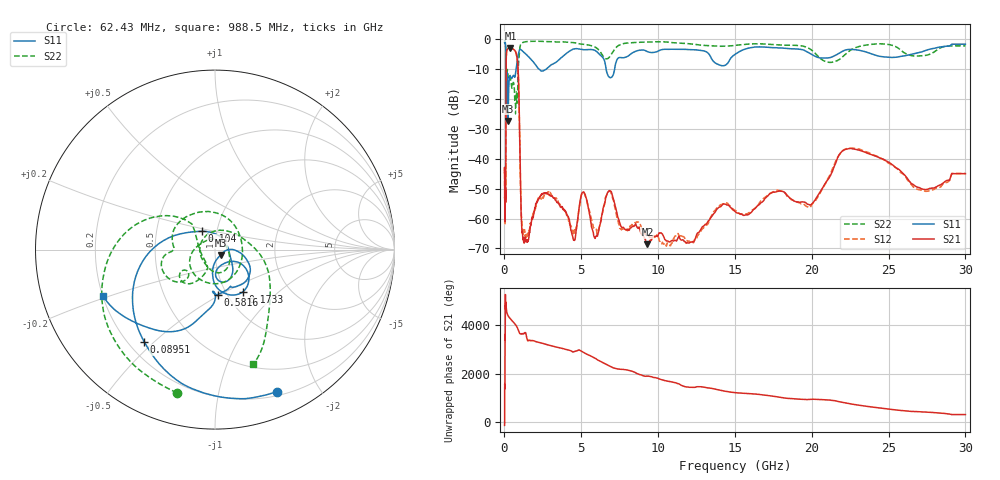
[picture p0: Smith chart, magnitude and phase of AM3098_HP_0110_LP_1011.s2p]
! Date/Time: Thu, Feb 28, 2019 8:37 AM
! Network Analyzer: Agilent Technologies E8364B Rev: A.07.50.67
! Sweep from 0.010 to 30.000 GHz, 1601 Points, Sweep Type: LOG
! Power Supply: 5.023 V, 0.002 A
# Hz S DB R 50
!freq MagS11 AngS11 MagS21 AngS21 MagS12 AngS12 MagS22 AngS22
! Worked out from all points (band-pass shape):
!   1601 points, 10 MHz to 30 GHz, reference 50 ohm
!   highest |S21| = -2.82 dB at 387.8 MHz (marker M1); lowest = -68.7 dB at 9.302 GHz (marker M2)
!   |S21| within 3 dB of the highest: 118.3 MHz to 807.5 MHz (689.2 MHz wide, 149 % of centre)
!   lowest |S11| = -27.4 dB at 237.5 MHz (marker M3), VSWR 1.09, Z = 53.1 - j3.16 ohm
!   |S11| at or under -10 dB: 99.92 MHz to 756.9 MHz (657 MHz wide, 153 % of centre); 2.273 GHz to 2.707 GHz (434.2 MHz wide, 17.4 % of centre); 6.618 GHz to 7.169 GHz (550.4 MHz wide, 7.98 % of centre)
!   |S22| runs from -24.9 to -0.6 dB; largest |S21 - S12| = 0.012
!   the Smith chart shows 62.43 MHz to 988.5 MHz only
!   S11 on the Smith chart (normalised r, x): 62.43 MHz: 0.24, -1.50; 89.51 MHz: 0.26, -0.46; 104 MHz: 0.85, +0.18; 173.3 MHz: 1.19, -0.61; 581.6 MHz: 0.91, -0.48; 988.5 MHz: 0.20, -0.19
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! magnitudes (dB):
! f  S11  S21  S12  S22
! 10 MHz  -0.3  -44.7  -44.0  -0.6
! 38.04 MHz  -0.5  -60.5  -61.3  -1.0
! 62.43 MHz  -1.3  -51.8  -51.6  -1.7
! 89.51 MHz  -3.8  -41.0  -40.9  -4.1
! 104 MHz  -18.1  -12.6  -12.6  -21.1
! 144.7 MHz  -18.8  -3.9  -3.8  -14.0
! 173.3 MHz  -11.0  -3.5  -3.5  -10.3
! 237.5 MHz  -27.4  -2.9  -2.9  -12.4
! 387.8 MHz  -12.4  -2.8  -2.8  -12.9
! 550.5 MHz  -12.3  -3.2  -3.2  -14.6
! 581.6 MHz  -12.0  -3.3  -3.2  -14.4
! 859.3 MHz  -6.3  -8.1  -8.1  -17.6
! 988.5 MHz  -3.4  -32.7  -32.6  -3.4
! 1.232 GHz  -4.2  -67.5  -63.8  -1.0
! 2.084 GHz  -8.9  -54.8  -55.4  -0.6
! 5.929 GHz  -3.8  -66.2  -63.5  -2.6
! 6.855 GHz  -12.8  -50.6  -50.8  -5.7
! 7.926 GHz  -5.9  -63.8  -63.9  -1.2
! 9.302 GHz  -4.1  -68.7  -65.5  -0.9
! 19.7 GHz  -4.2  -55.2  -56.1  -2.7
! 22.67 GHz  -3.4  -36.7  -36.4  -3.1
! 30 GHz  -1.6  -45.0  -44.9  -2.2
